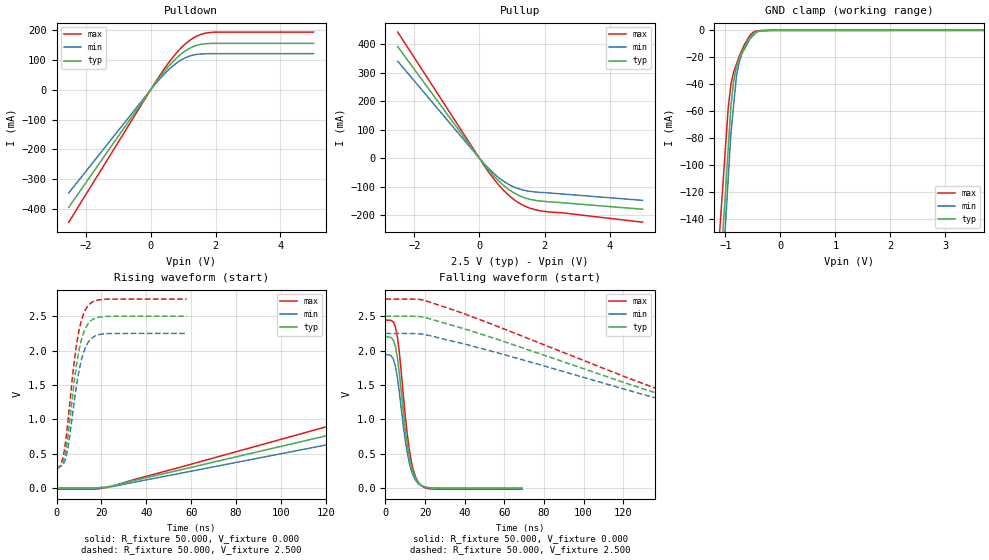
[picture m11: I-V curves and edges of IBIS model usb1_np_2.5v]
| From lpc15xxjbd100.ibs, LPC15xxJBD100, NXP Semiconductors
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[Model]   usb1_np_2.5v
Model_type I/O
Vinl=8.000E-01
Vinh=1.750E+00
Vref=0.000E+00
Rref=1.000E+06
Cref=0.000E+00
Vmeas=1.250E+00
C_comp   2.000E-12   2.000E-12   2.000E-12
[Voltage Range]   2.500E+00   2.250E+00   2.750E+00
[POWER Clamp Reference]   2.500E+00   2.250E+00   2.750E+00
[GND Clamp Reference]   0.000E+00   0.000E+00   0.000E+00
[Pullup Reference]   2.500E+00   2.250E+00   2.750E+00
[Pulldown Reference]   0.000E+00   0.000E+00   0.000E+00
[Temperature Range]   25   85   -40
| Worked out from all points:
|   slope of the pulldown table from 0 to 0.375 V, typ, clamps not added: 6.8 ohm
|   slope of the pullup table from 0 to 0.375 V, typ, clamps not added: 6.99 ohm
|   GND clamp passes 1 mA (typ) near -0.43 V on its own axis
|   rising waveform, R_fixture 50.000, V_fixture 0.000: 20-80 % time 190ns typ, 204ns min, 177ns max; typ from 0 V to 2.2 V
|   falling waveform, R_fixture 50.000, V_fixture 0.000: 20-80 % time 5.54ns typ, 5.62ns min, 5.44ns max; typ from 2.2 V to 0 V
|   rising waveform, R_fixture 50.000, V_fixture 2.500: 20-80 % time 5.36ns typ, 5.45ns min, 5.37ns max; typ from 0.301 V to 2.5 V
|   falling waveform, R_fixture 50.000, V_fixture 2.500: 20-80 % time 143ns typ, 150ns min, 137ns max; typ from 2.5 V to 0.301 V
[GND Clamp]
-2.5V     -1.085A    -1.161A    -972.7mA
-950mV    -88.05mA   -110.3mA   -57.74mA
-900mV    -55.88mA   -76.4mA    -40.03mA
-850mV    -37.37mA   -55.15mA   -30.87mA
-800mV    -27.05mA   -33.9mA    -25.02mA
-750mV    -20.67mA   -23.6mA    -19.17mA
-700mV    -16.45mA   -17.38mA   -14.68mA
-600mV    -8.024mA   -9.842mA   -6.833mA
-500mV    -2.653mA   -3.954mA   -1.548mA
-400mV    -614.5uA   -826.9uA   -269.7uA
-150mV    -32.49uA   -28.84uA   -4.96uA
5V        18.49uA    17.79uA    3.905uA
[Power Clamp]
-2.51V    0A         0A         0A
0V        0A         0A         0A
2.5V      0A         0A         0A
5V        0A         0A         0A
[Pullup]
-2.51V    392.3mA    340.9mA    443.4mA
230mV     -33.95mA   -29.9mA    -40.38mA
470mV     -65.73mA   -56.29mA   -76.87mA
690mV     -90.27mA   -76.71mA   -106.7mA
1.05V     -121.1mA   -100.7mA   -144.5mA
1.43V     -140.7mA   -114.1mA   -170.1mA
1.85V     -150.2mA   -119.8mA   -184.3mA
5.01V     -179.1mA   -148.1mA   -224.8mA
[Pulldown]
-2.52V    -393.9mA   -345.8mA   -444.1mA
160mV     24.62mA    21.35mA    27.98mA
480mV     69.42mA    59.44mA    79.66mA
740mV     100.4mA    84.72mA    116.4mA
960mV     122.2mA    101.4mA    143.1mA
1.18V     138.2mA    112.6mA    163.8mA
1.5V      151.7mA    119.9mA    184.1mA
1.88V     155.9mA    121.4mA    193mA
5.02V     156.1mA    121.5mA    193.9mA
[Rising Waveform]
R_fixture = 50.000
V_fixture = 0.000
V_fixture_min = 0.000
V_fixture_max = 0.000
|  time   V(typ)   V(min)   V(max)
0s        175.6uV    175.7uV    -15.47mV
23ns      19.77mV    13.13mV    12.49mV
124ns     788.9mV    651.3mV    925.5mV
194ns     1.295V     1.073V     1.52V
253ns     1.675V     1.393V     1.961V
291ns     1.872V     1.571V     2.169V
338ns     2.023V     1.728V     2.304V
400ns     2.12V      1.841V     2.381V
472ns     2.168V     1.902V     2.418V
586ns     2.198V     1.941V     2.441V
[Falling Waveform]
R_fixture = 50.000
V_fixture = 0.000
V_fixture_min = 0.000
V_fixture_max = 0.000
|  time   V(typ)   V(min)   V(max)
0s        2.198V     1.941V     2.442V
3ns       2.188V     1.921V     2.438V
5ns       2.063V     1.774V     2.348V
7ns       1.669V     1.393V     1.973V
10ns      853.6mV    693mV      1.048V
12ns      460.5mV    371.5mV    563.7mV
14ns      226.4mV    183mV      269mV
17ns      67.55mV    56.11mV    67.14mV
24ns      2.729mV    2.6mV      -12.71mV
69ns      175.6uV    175.7uV    -14.78mV
[Rising Waveform]
R_fixture = 50.000
V_fixture = 2.500
V_fixture_min = 2.250
V_fixture_max = 2.750
|  time   V(typ)   V(min)   V(max)
0s        301.1mV    307.8mV    293.6mV
2ns       319.4mV    314.6mV    344.4mV
3ns       378.4mV    343.9mV    455.6mV
4ns       512.9mV    421.8mV    658.3mV
6ns       1.006V     780.7mV    1.267V
9ns       1.811V     1.514V     2.108V
11ns      2.147V     1.856V     2.429V
14ns      2.388V     2.117V     2.651V
21ns      2.495V     2.243V     2.746V
58ns      2.5V       2.25V      2.75V
[Falling Waveform]
R_fixture = 50.000
V_fixture = 2.500
V_fixture_min = 2.250
V_fixture_max = 2.750
|  time   V(typ)   V(min)   V(max)
0s        2.5V       2.25V      2.75V
17ns      2.496V     2.244V     2.745V
31ns      2.39V      2.157V     2.623V
165ns     1.126V     1.091V     1.149V
210ns     740.3mV    762.6mV    703.4mV
233ns     570.3mV    612.1mV    520.4mV
259ns     443.1mV    482.3mV    404.8mV
292ns     365.9mV    390.3mV    342mV
334ns     323.3mV    336.5mV    310.2mV
393ns     301.1mV    307.8mV    293.6mV
[Ramp]
dV/dt_r   1.3136E+00/1.8912E-07   1.1585E+00/2.0389E-07   1.4741E+00/1.7664E-07
dV/dt_f   1.3193E+00/1.4271E-07   1.1653E+00/1.4991E-07   1.4738E+00/1.3645E-07
R_load = 50
